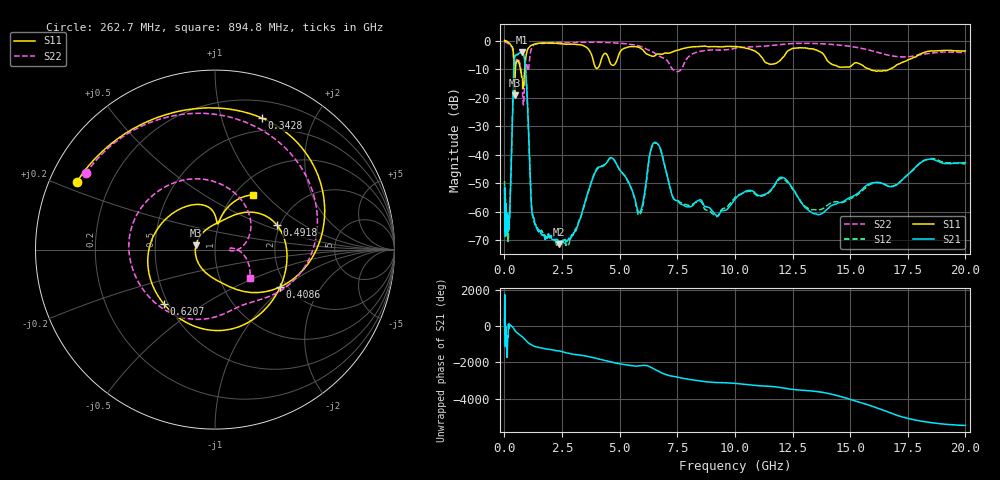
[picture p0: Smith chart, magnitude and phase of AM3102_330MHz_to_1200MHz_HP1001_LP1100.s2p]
! Date/Time: Tue, Sep 11, 2018 5:18 PM
! Network Analyzer: Agilent Technologies E8362B Rev: A.07.50.63
! Sweep from 0.010 to 20.000 GHz, 1601 Points, Sweep Type: LOG
! Power Supply: 4.949 V, 0.001 A
# Hz S DB R 50
!freq MagS11 AngS11 MagS21 AngS21 MagS12 AngS12 MagS22 AngS22
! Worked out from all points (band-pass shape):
!   1601 points, 10 MHz to 20 GHz, reference 50 ohm
!   highest |S21| = -4.18 dB at 754.2 MHz (marker M1); lowest = -71.4 dB at 2.381 GHz (marker M2)
!   |S21| within 3 dB of the highest: 428.9 MHz to 884.3 MHz (455.5 MHz wide, 69.4 % of centre)
!   lowest |S11| = -19.2 dB at 443 MHz (marker M3), VSWR 1.24, Z = 40.4 + j2.02 ohm
!   |S11| at or under -10 dB: 416.2 MHz to 477.8 MHz (61.59 MHz wide, 13.8 % of centre); 696.4 MHz to 881.4 MHz (185 MHz wide, 23.5 % of centre); 15.84 GHz to 16.73 GHz (896.7 MHz wide, 5.51 % of centre)
!   |S22| runs from -22.6 to -0.2 dB; largest |S21 - S12| = 0.0099
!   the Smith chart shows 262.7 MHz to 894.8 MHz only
!   S11 on the Smith chart (normalised r, x): 262.7 MHz: 0.08, +0.23; 342.8 MHz: 0.36, +1.35; 408.6 MHz: 1.83, -0.93; 491.8 MHz: 1.92, +0.61; 620.7 MHz: 0.48, -0.35; 894.8 MHz: 1.20, +0.85
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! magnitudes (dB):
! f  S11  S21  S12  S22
! 10 MHz  0.0  -59.5  -49.7  -0.2
! 35.55 MHz  0.0  -64.2  -65.9  -0.5
! 126.4 MHz  -0.4  -66.0  -65.8  -0.9
! 168.9 MHz  -0.6  -65.4  -68.1  -1.1
! 262.7 MHz  -1.3  -53.4  -53.6  -1.6
! 342.8 MHz  -2.2  -29.3  -29.4  -2.7
! 408.6 MHz  -7.6  -10.5  -10.5  -6.2
! 443 MHz  -19.2  -6.0  -6.1  -9.2
! 447.2 MHz  -19.0  -5.8  -5.8  -9.2
! 491.8 MHz  -8.6  -5.1  -5.1  -7.6
! 620.7 MHz  -7.6  -4.5  -4.7  -6.8
! 754.2 MHz  -12.8  -4.2  -4.2  -13.1
! 894.8 MHz  -8.6  -7.9  -8.0  -12.0
! 1.201 GHz  -1.6  -60.4  -60.6  -2.3
! 1.59 GHz  -1.0  -67.6  -66.9  -0.9
! 2.381 GHz  -1.1  -71.4  -71.1  -0.7
! 4.564 GHz  -7.3  -41.5  -41.3  -0.7
! 5.652 GHz  -2.1  -55.2  -55.6  -1.6
! 6.549 GHz  -5.2  -35.8  -36.0  -4.6
! 7.517 GHz  -3.4  -56.3  -56.2  -10.9
! 9.047 GHz  -2.1  -60.0  -60.9  -3.3
! 20 GHz  -3.6  -42.8  -43.3  -4.2
